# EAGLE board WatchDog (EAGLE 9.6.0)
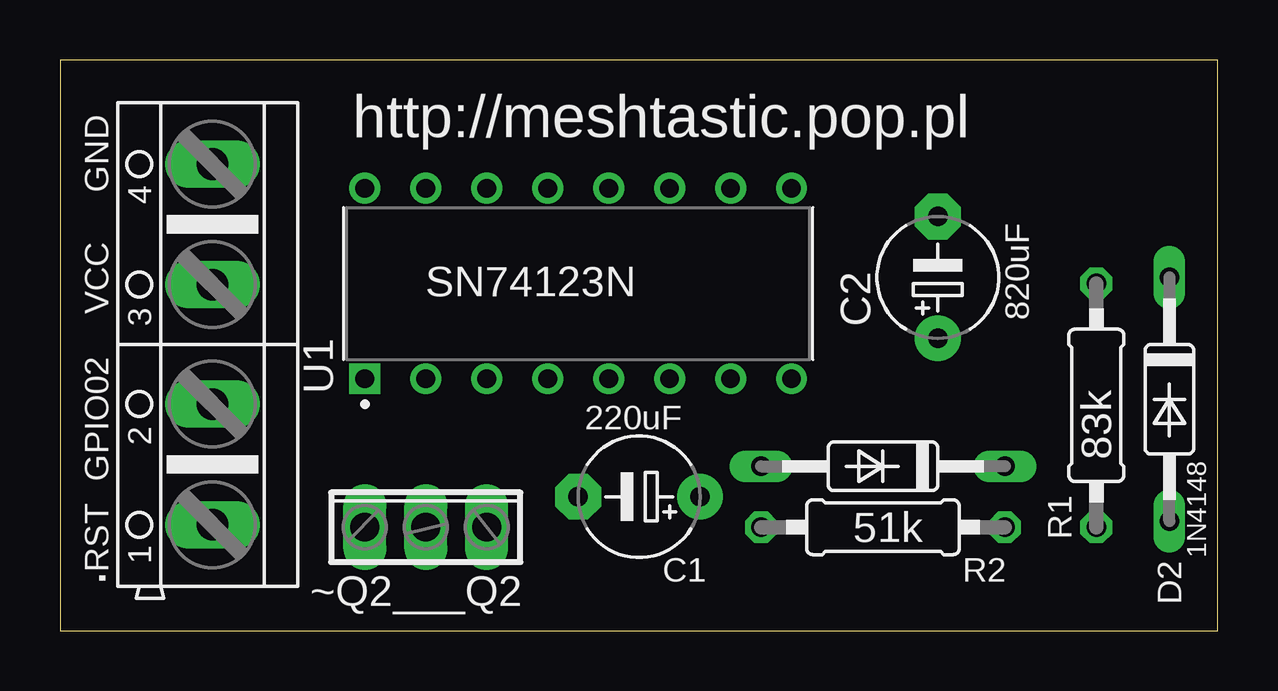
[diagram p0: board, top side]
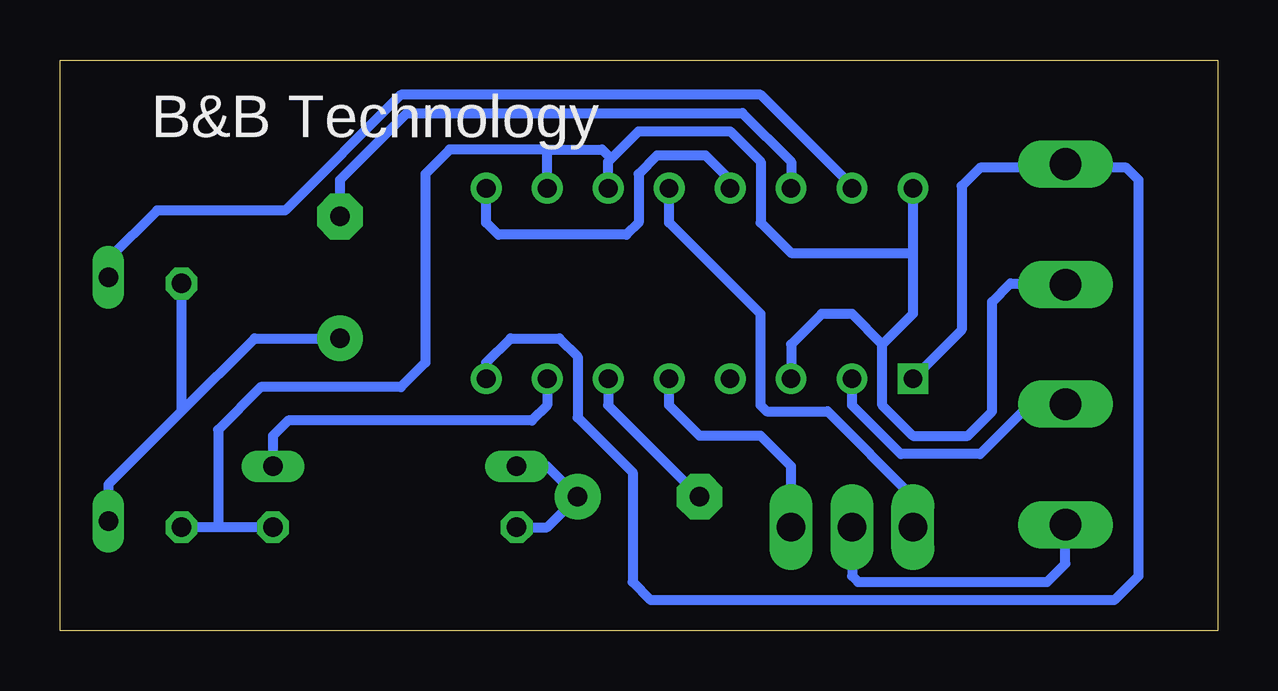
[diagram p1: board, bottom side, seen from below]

Size 48.24 x 23.8 mm. Coordinates in mm from the lower left corner, seen from the top.
Outline: 0,0 48.24,0 48.24,23.8 0,23.8 0,0
Copper layers (1*16): Top 0.035mm / dielectric 1.5mm / Bottom 0.035mm
Design rules "default": minimum track width 10mil, minimum drill 24mil, track to track 8mil, track to pad 8mil, pad to pad 8mil, via to via 8mil, smd to smd 8mil, copper to edge 40mil, drill to drill 8mil, minimum pad ring 10mil, minimum via ring 8mil, stop-mask expansion 4mil, vias tented up to drill 0mil, thermal gap 10mil

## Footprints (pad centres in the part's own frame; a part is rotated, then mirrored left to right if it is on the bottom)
AK500/4 = drill 1.321 long: 1 -7.518,0; 2 -2.489,0; 3 2.489,0; 4 7.518,0
E5-5 = drill 0.813 pad 1.905: + -2.54,0 | drill 0.813 pad 1.905 octagon: - 2.54,0
DO35-10 = drill 0.813 long: A 5.08,0; C -5.08,0
0207/10 = drill 0.813 octagon: 1 -5.08,0; 2 5.08,0
DIP794W45P254L1969H508Q16 = drill 0.78 pad 1.13 square: 1 -3.97,8.89 | drill 0.78 pad 1.13: 2 -3.97,6.35; 3 -3.97,3.81; 4 -3.97,1.27; 5 -3.97,-1.27; 6 -3.97,-3.81; 7 -3.97,-6.35; 8 -3.97,-8.89; 9 3.97,-8.89; 10 3.97,-6.35; 11 3.97,-3.81; 12 3.97,-1.27; 13 3.97,1.27; 14 3.97,3.81; 15 3.97,6.35; 16 3.97,8.89
3POL254 = drill 1.2 long: 1 -2.54,0; 2 0,0; 3 2.54,0

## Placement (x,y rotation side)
.  [AK500/4]  6.35,11.94 90 top
C1  220uF  [E5-5]  24.13,5.59 180 top
C2  820uF  [E5-5]  36.58,14.73 90 top
D1  1N4148  [DO35-10]  34.29,6.86 180 top
D2  1N4148DO35-10  [DO35-10]  46.23,9.65 270 top
R1  83k  [0207/10]  43.18,9.4 90 top
R2  51k  [0207/10]  34.29,4.32 0 top
U1  SN74123N  [DIP794W45P254L1969H508Q16]  21.59,14.48 90 top
~Q2___Q2  [3POL254]  15.24,4.32 0 top

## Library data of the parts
. = con-ptr500; OC_FARNELL: unknown; OC_NEWARK: unknown
C1 C2 = rcl
D1 D2 = diode
R1 R2 = resistor
U1 = sn74123n; AVAILABILITY: In Stock; CHECK_PRICES: https://www.snapeda.com/parts/SN74123N/Texas+Instruments/view-part/?ref=eda; DESCRIPTION: Dual retriggerable monostable multivibrators; MF: Texas Instruments; MP: SN74123N; PACKAGE: PDIP-16 Texas Instruments; PRICE: None; PURCHASE-URL: https://www.snapeda.com/api/url_track_click_mouser/?unipart_id=301413&manufacturer=Texas Instruments&part_name=SN74123N&search_term=None; SNAPEDA_LINK: https://www.snapeda.com/parts/SN74123N/Texas+Instruments/view-part/?ref=snap
~Q2___Q2 = con-phoenix-254; OC_FARNELL: unknown; OC_NEWARK: unknown

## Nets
B1: ..2 U1.2
GND: ..4 U1.1 U1.8
N$1: C2.+ D2.A R1.2
N$2: D2.C U1.15
N$3: ..1 ~Q2___Q2.2
N$4: C1.- U1.6
N$8: C1.+ D1.A R2.1
N$9: D1.C U1.7
N$10: C2.- U1.14
Q2: U1.5 ~Q2___Q2.3
VCC: ..3 R1.1 R2.2 U1.3 U1.10 U1.11 U1.16
ZW: U1.9 U1.13
~Q2: U1.12 ~Q2___Q2.1

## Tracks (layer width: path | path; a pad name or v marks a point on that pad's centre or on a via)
B1
  Bottom 0.406: ..2 7.82,9.45 9.91,7.37 13.21,7.37 15.24,9.4 U1.2
GND
  Bottom 0.406: U1.1 10.67,12.54 10.67,18.54 9.91,19.3 6.2,19.3 | U1.8 30.48,11.18 29.46,12.19 27.43,12.19 26.67,11.43 26.67,8.89 24.38,6.6 24.38,2.03 23.62,1.27 4.32,1.27 3.3,2.29 3.3,18.8 3.81,19.3 6.2,19.3 | 6.2,19.3 ..4
N$1
  Bottom 0.406: 43.18,9.14 40.13,12.19 C2.+ | 43.18,9.14 46.23,6.1 D2.A | R1.2 43.18,9.14
N$2
  Bottom 0.406: U1.15 15.24,18.54 19.05,22.35 34.04,22.35 38.86,17.53 44.2,17.53 46.23,15.49 D2.C
N$3
  Bottom 0.406: ~Q2___Q2.2 15.24,2.29 14.99,2.03 7.11,2.03 6.35,2.79 ..1
N$4
  Bottom 0.406: U1.6 25.4,9.4 C1.-
N$8
  Bottom 0.406: R2.1 27.94,4.32 C1.+ 27.94,6.86 D1.A
N$9
  Bottom 0.406: U1.7 27.94,9.4 28.58,8.76 38.73,8.76 39.37,8.13 D1.C
N$10
  Bottom 0.406: U1.14 17.78,19.56 19.81,21.59 33.78,21.59 36.58,18.8 C2.-
Q2
  Bottom 0.406: ~Q2___Q2.3 17.78,6.86 19.05,8.13 21.59,8.13 22.86,9.4 U1.5
VCC
  Bottom 0.406: 13.97,11.94 13.97,9.4 12.7,8.13 10.41,8.13 9.4,9.14 9.4,13.72 8.64,14.48 6.4,14.48 ..3 | 13.97,11.94 15.24,13.21 16.51,13.21 17.78,11.94 U1.3 | U1.16 12.7,15.75 | 12.7,15.75 12.7,13.21 13.97,11.94 | R2.2 41.66,4.32 | 41.66,4.32 R1.1 | U1.11 25.4,19.56 25.27,19.68 | 25.27,19.68 24.13,20.83 20.32,20.83 19.05,19.56 19.05,17.02 17.78,15.75 12.7,15.75 | 27.94,20.07 25.65,20.07 25.27,19.68 | U1.10 27.94,20.07 | 27.94,20.07 32,20.07 33.02,19.05 33.02,11.18 34.04,10.16 39.88,10.16 41.66,8.38 41.66,4.32
ZW
  Bottom 0.406: U1.13 20.32,18.8 21.34,19.81 23.37,19.81 24.13,19.05 24.13,17.02 24.64,16.51 29.97,16.51 30.48,17.02 U1.9
~Q2
  Bottom 0.406: U1.12 22.86,17.02 19.05,13.21 19.05,9.4 18.8,9.14 16.26,9.14 12.7,5.59 ~Q2___Q2.1

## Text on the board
tPlace: GND | VCC | GPIO02 | RST
tNames: http://meshtastic.pop.pl | 1N4148
bNames: B&B Technology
